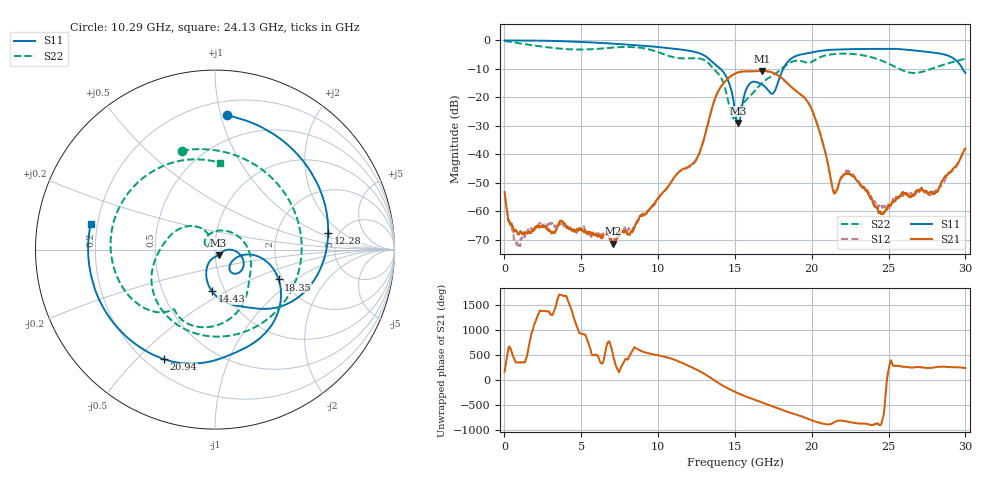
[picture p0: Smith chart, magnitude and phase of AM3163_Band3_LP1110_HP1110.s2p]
!Agilent Technologies,E8364B,MY43040894,A.07.50.67
!Agilent E8364B: A.07.50.67
!Date: Thursday, August 20, 2020 11:07:06
!Correction: S11(Full 2 Port(1,2))
!S21(Full 2 Port(1,2))
!S12(Full 2 Port(1,2))
!S22(Full 2 Port(1,2))
!S2P File: Measurements: S11, S21, S12, S22:
# Hz S  dB  R 50
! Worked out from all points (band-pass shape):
!   3201 points, 10 MHz to 30 GHz, reference 50 ohm
!   highest |S21| = -10.75 dB at 16.77 GHz (marker M1); lowest = -71.5 dB at 7.067 GHz (marker M2)
!   |S21| within 3 dB of the highest: 14.48 GHz to 18.16 GHz (3.677 GHz wide, 22.5 % of centre)
!   lowest |S11| = -29.0 dB at 15.21 GHz (marker M3), VSWR 1.07, Z = 51.9 - j3.04 ohm
!   |S11| at or under -10 dB: 14.06 GHz to 18.14 GHz (4.082 GHz wide, 25.4 % of centre); 29.82 GHz to end of sweep
!   |S22| runs from -27.4 to -0.2 dB; largest |S21 - S12| = 0.0051
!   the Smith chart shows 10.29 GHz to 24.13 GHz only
!   S11 on the Smith chart (normalised r, x): 10.29 GHz: 0.31, +1.05; 12.28 GHz: 4.10, +1.25; 14.43 GHz: 0.87, -0.42; 18.35 GHz: 1.91, -0.75; 20.94 GHz: 0.27, -0.60; 24.13 GHz: 0.17, +0.10
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1e7  -0.03 -1.9  -53.29 162.1  -55.74 72.3  -0.17 -5.2
1.218972e9  -0.05 -32.4  -67.88 -5.1  -68.96 15.4  -1.26 -82.6
2.624753e9  -0.14 -69.4  -65.70 -57.0  -64.92 -57.0  -2.32 -163.3
5.014581e9  -0.57 -130.0  -66.33 -154.8  -66.76 -165.1  -3.23 72.1
7.067022e9  -1.15 178.3  -71.49 138.0  -69.99 -15.8  -2.54 -40.7
8.294738e9  -1.60 145.6  -67.21 -154.0  -67.07 -28.1  -2.33 -112.1
1.000979e10  -2.34 94.3  -55.40 130.6  -55.87 133.7  -4.16 131.3
1.029095e10  -2.49 84.9  -53.53 111.5  -53.65 109.7  -4.71 108.5
1.132185e10  -3.10 48.0  -46.37 10.9  -46.52 10.6  -6.24 16.9
1.227778e10  -3.92 8.2  -43.21 -120.4  -43.67 -119.7  -6.26 -67.3
1.443332e10  -12.72 -94.5  -14.01 -155.1  -13.84 -154.6  -18.30 118.5
1.5005e10  -25.10 -108.8  -11.69 118.0  -11.64 118.2  -27.22 150.4
1.521118e10  -29.04 -55.8  -11.25 89.1  -11.22 89.5  -25.01 156.4
1.676691e10  -15.55 -52.7  -10.75 -94.6  -10.67 -94.8  -14.98 5.9
1.835076e10  -8.15 -25.1  -14.71 84.1  -14.79 84.8  -8.62 -70.8
2.000958e10  -4.24 -89.2  -24.40 -94.7  -24.29 -94.1  -7.52 -126.1
2.09374e10  -3.43 -115.1  -40.59 -172.5  -40.37 -170.7  -5.23 -153.1
2.147159e10  -3.26 -128.9  -53.83 -131.1  -53.31 -140.2  -4.82 -171.5
2.413321e10  -3.01 168.5  -58.50 -159.5  -57.13 157.1  -6.31 86.8
2.500479e10  -3.05 147.2  -57.83 -153.5  -58.93 29.6  -8.21 43.1
2.715095e10  -3.82 87.7  -51.75 -108.8  -52.47 -113.9  -11.12 -101.4
3e10  -11.45 -21.9  -38.04 -124.5  -38.01 -124.9  -6.42 126.6
